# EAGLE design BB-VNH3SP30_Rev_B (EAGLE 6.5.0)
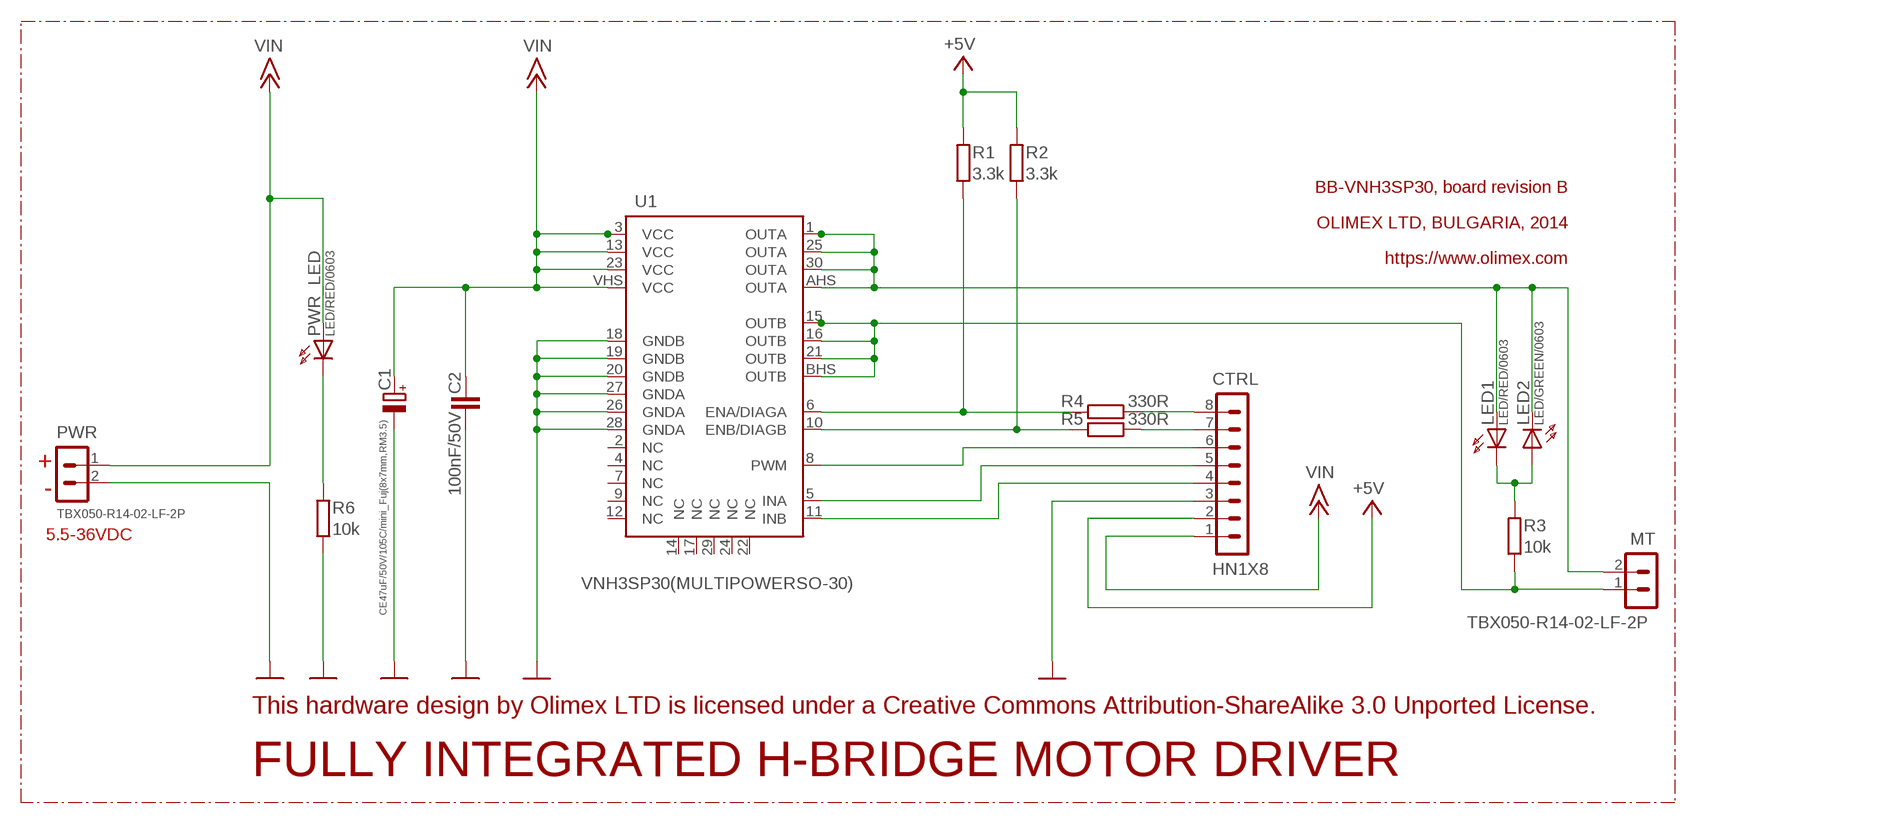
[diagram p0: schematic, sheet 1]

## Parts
C1  CE47uF/50V/105C/mini_Fuj(8x7mm,RM3.5)  CPOL-EUE3.5-8  [E3,5-8]
C2  100nF/50V  C-EUC0603_DWS  [C0603_DWS]
CTRL  HN1X8  CON8HN1X8  [HN1X8]
LED1  LED/RED/0603  LED0603DWS  [LED-0603]
LED2  LED/GREEN/0603  LED0603DWS  [LED-0603]
MT  TBX050-R14-02-LF-2P  CON2_TBX050-R14-02-LF-2P  [TBX050-R14-02-LF-2P]
PWR  TBX050-R14-02-LF-2P  CON2_TBX050-R14-02-LF-2P  [TBX050-R14-02-LF-2P]
PWR_LED  LED/RED/0603  LED0603DWS  [LED-0603]
R1  3.3k  R-EU_R0603_5MIL_DWS  [R0603_5MIL_DWS]
R2  3.3k  R-EU_R0603_5MIL_DWS  [R0603_5MIL_DWS]
R3  10k  R-EU_R0603_5MIL_DWS  [R0603_5MIL_DWS]
R4  330R  R-EU_R0603_5MIL_DWS  [R0603_5MIL_DWS]
R5  330R  R-EU_R0603_5MIL_DWS  [R0603_5MIL_DWS]
R6  10k  R-EU_R0603_5MIL_DWS  [R0603_5MIL_DWS]
U1  VNH3SP30(MULTIPOWERSO-30)  [MULTIPOWERSO-30]

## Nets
+5V: CTRL.2 R1.2 R2.2
+15V: C1.+ C2.2 CTRL.1 PWR.1 PWR_LED.A U1.3(VCC) U1.13(VCC) U1.23(VCC) U1.VHS1 U1.VHS2 U1.VHS3 U1.VHS4 U1.VHS5 U1.VHS6 U1.VHS7 U1.VHS8 U1.VHS9 U1.VHS10 U1.VHS11 U1.VHS(VCC) ; supply symbol labelled VIN
GND [pwr]: C1.- C2.1 CTRL.3 PWR.2 R6.1 U1.18(GNDB) U1.19(GNDB) U1.20(GNDB) U1.26(GNDA) U1.27(GNDA) U1.28(GNDA)
N$1: R1.1 R4.2 U1.6(ENA/DIAGA)
N$2: LED1.C LED2.A R3.2
N$3: CTRL.8 R4.1
N$4: CTRL.7 R5.1
N$5: PWR_LED.C R6.2
N$9: CTRL.6 U1.8(PWM)
N$10: R2.1 R5.2 U1.10(ENB/DIAGB)
N$11: CTRL.5 U1.5(INA)
N$16: CTRL.4 U1.11(INB)
OUTA: LED1.A LED2.C MT.2 U1.1(OUTA) U1.25(OUTA) U1.30(OUTA) U1.AHS1 U1.AHS2 U1.AHS3 U1.AHS4 U1.AHS5 U1.AHS(OUTA)
OUTB: MT.1 R3.1 U1.15(OUTB) U1.16(OUTB) U1.21(OUTB) U1.BHS1 U1.BHS2 U1.BHS3 U1.BHS4 U1.BHS5 U1.BHS(OUTB)
Unconnected: U1.2(NC) U1.4(NC) U1.7(NC) U1.9(NC) U1.12(NC) U1.14(NC) U1.17(NC) U1.22(NC) U1.24(NC) U1.29(NC)

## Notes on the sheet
- BB-VNH3SP30, board revision B
- OLIMEX LTD, BULGARIA, 2014
- https://www.olimex.com
- +
- -
- 5.5-36VDC
- This hardware design by Olimex LTD is licensed under a Creative Commons Attribution-ShareAlike 3.0 Unported License.
- FULLY INTEGRATED H-BRIDGE MOTOR DRIVER

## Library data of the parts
C1 = rcl:CPOL-EU: POLARIZED CAPACITOR, European symbol
C2 = rcl:C-EU: CAPACITOR, European symbol
CTRL = Penko:CON8
LED1 LED2 PWR_LED = DOUBLE-SIDE:LED
MT PWR = Penko:CON2
R1-R6 = rcl:R-EU_: RESISTOR, European symbol
U1 = OLIMEX_IC:VNH3SP30: VNH3SP30 FULLY INTEGRATED H-BRIDGE MOTOR DRIVER

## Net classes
0 default: width 0.254 mm, drill 0.6 mm, clearance 0.254 mm
1 pwr: width 0.25 mm
2 thin: width 0.025 mm, clearance 0.025 mm
3 gsm_pwr: width 0.914 mm, drill 0.787 mm

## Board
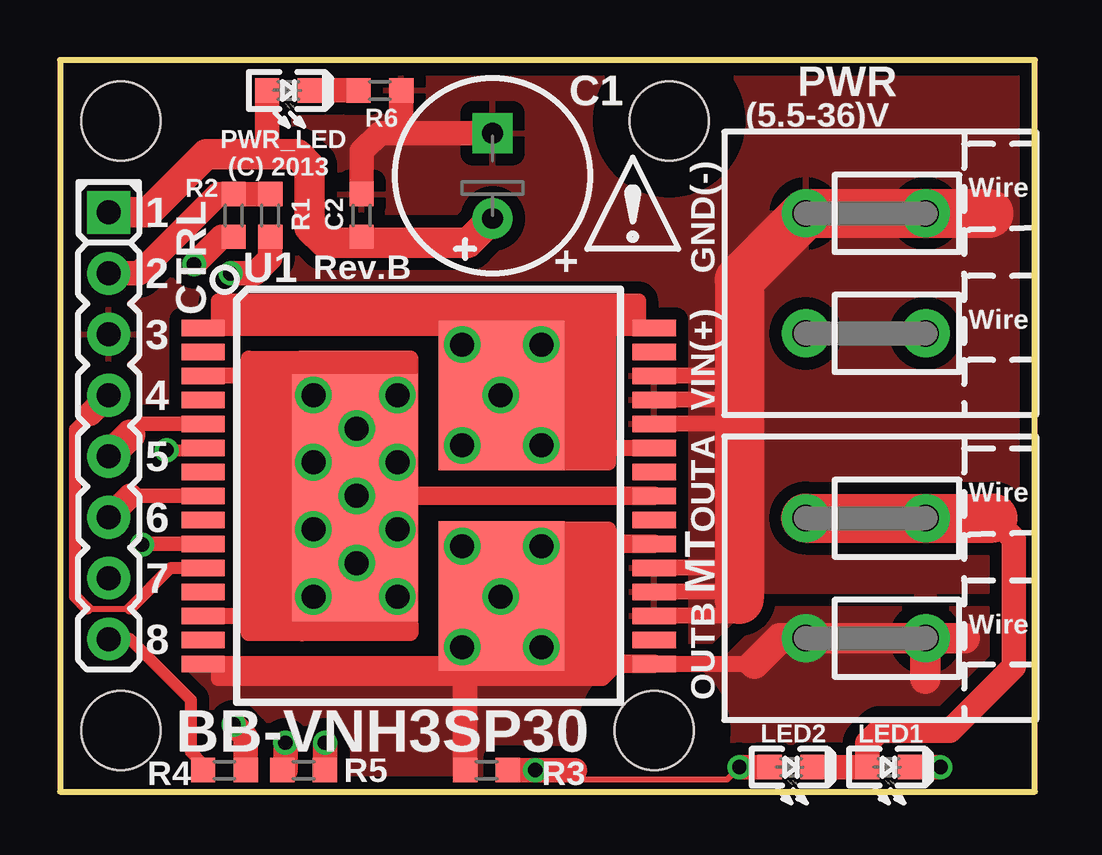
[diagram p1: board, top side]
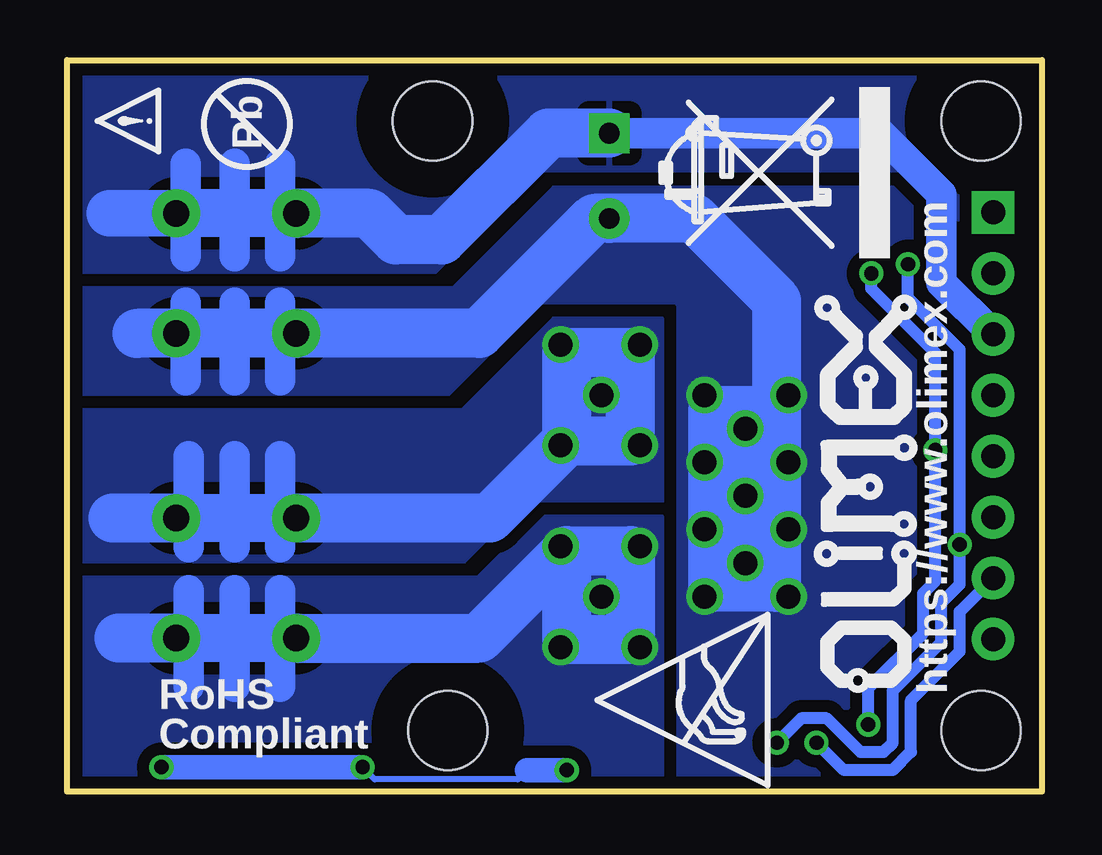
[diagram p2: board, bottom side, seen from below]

Size 40.64 x 30.48 mm. Coordinates in mm from the lower left corner, seen from the top.
Outline: 0,0 40.64,0 40.64,30.48 0,30.48 0,0
Copper layers (1+16): Top 0.035mm / dielectric 1.5mm / Bottom 0.035mm
Design rules "default": minimum track width 9.5mil, minimum drill 23mil, track to track 9.5mil, track to pad 9.5mil, pad to pad 9.5mil, via to via 10mil, smd to smd 1mil, copper to edge 10mil, drill to drill 8mil, minimum pad ring 10mil, minimum via ring 8mil, stop-mask expansion 4mil, vias tented up to drill 25mil, thermal gap 20mil
Holes 3.3 mm at 2.54,27.94 25.4,27.94 24.77,2.54 2.54,2.54
tRestrict: area 0,0 to 5.1,5.1; area 22.2,0 to 27.3,5.1; area 22.9,25.4 to 27.9,30.5; area 0,25.4 to 5.1,30.5
bRestrict: area 0,25.4 to 5.1,30.5; area 22.9,25.4 to 27.9,30.5; area 0,0 to 5.1,5.1; area 22.2,0 to 27.3,5.1

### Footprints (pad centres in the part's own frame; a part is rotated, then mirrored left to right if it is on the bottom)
E3,5-8 = drill 0.864 pad 1.676: + -1.778,0 | drill 0.864 pad 1.676 square: - 1.778,0
C0603_DWS = smd 1.016 x 1.016: 1 -0.889,0; 2 0.889,0
HN1X8 = drill 1 pad 1.778 square: 1 -8.89,0 | drill 1 pad 1.778: 2 -6.35,0; 3 -3.81,0; 4 -1.27,0; 5 1.27,0; 6 3.81,0; 7 6.35,0; 8 8.89,0
LED-0603 = smd 1.016 x 1.016: A 0.889,0; C -0.889,0
TBX050-R14-02-LF-2P = drill 1.1 pad 2: 1 -2.5,3.2; 2 2.5,3.2; 3 -2.5,-1.8; 4 2.5,-1.8
R0603_5MIL_DWS = smd 1.016 x 1.016: 1 -0.889,0; 2 0.889,0
MULTIPOWERSO-30 = smd 0.68 x 1.8: 1 -7,-9.4; 2 -6,-9.4; 3 -5,-9.4; 4 -4,-9.4; 5 -3,-9.4; 6 -2,-9.4; 7 -1,-9.4; 8 0,-9.4; 9 1,-9.4; 10 2,-9.4; 11 3,-9.4; 12 4,-9.4; 13 5,-9.4; 14 6,-9.4; 15 7,-9.4; 16 7,9.4; 17 6,9.4; 18 5,9.4; 19 4,9.4; 20 3,9.4; 21 2,9.4; 22 1,9.4; 23 0,9.4; 24 -1,9.4; 25 -2,9.4; 26 -3,9.4; 27 -4,9.4; 28 -5,9.4; 29 -6,9.4; 30 -7,9.4 | smd 6.23 x 5.25: AHS -4.173,3.049; BHS 4.163,3.047 | drill 1 pad 1.524: AHS1 -6.3,4.7; AHS2 -4.2,3; AHS3 -2.1,4.7; AHS4 -6.3,1.4; AHS5 -2.1,1.4; BHS1 2.1,4.7; BHS2 4.2,3; BHS3 6.3,4.7; BHS4 2.1,1.4; BHS5 6.3,1.4; VHS1 -4.2,-1.3; VHS2 -1.4,-1.3; VHS3 1.4,-1.3; VHS4 4.2,-1.3; VHS5 -4.2,-4.8; VHS6 -1.4,-4.8; VHS7 1.4,-4.8; VHS8 4.2,-4.8; VHS9 -2.8,-3; VHS10 0,-3; VHS11 2.8,-3 | smd 10.3 x 5.25: VHS 0.075,-3.055

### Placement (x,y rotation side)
C1  18.03,25.65 90 top
C2  12.57,24 270 top
CTRL  2.03,15.24 270 top
LED1  34.54,1.02 180 top
LED2  30.48,1.02 180 top
MT  34.29,8.89 90 top
PWR  34.29,21.59 90 top
PWR_LED  9.53,29.21 180 top
R1  8.76,24 90 top
R2  7.24,24 90 top
R3  17.78,0.89 0 top
R4  6.86,0.89 0 top
R5  10.16,0.89 0 top
R6  13.34,29.21 180 top
U1  15.37,12.32 270 top
U$1  [RECYCLE_BIN1/6]  6.35,22.23 90 bottom
U$2  [ATTENTION_SMALL]  36.83,26.67 90 bottom
U$3  [PB_SMALL]  33.15,27.81 90 bottom
U$4  [ATTENTION]  21.97,22.61 0 top
U$5  [ESD_SYMBOL]  11.43,0.25 90 bottom
U$14  [OLIMEX1_V]  5.08,21.84 90 bottom

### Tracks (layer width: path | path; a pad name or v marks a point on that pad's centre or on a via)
+5V
  Top 1.016: CTRL.2 3.3,21.59 6.6,24.89 R2.2 R1.2
+15V
  Top 0.61: 12.45,12.32 U1.VHS10 12.31,12.32 U1.VHS
  Top 0.66: 12.19,17.32 U1.3 | 12.19,12.24 12.19,17.32 | 12.19,12.24 U1.VHS | U1.13 9.91,7.32 | 9.91,7.32 12.19,7.32 12.19,12.24 | 9.91,7.32 10.03,7.32 10.03,6.99 | 10.03,6.99 10.03,6.6 10.16,6.6 | 10.16,6.6 14.61,6.6 14.61,6.99 10.03,6.99 | 12.19,17.32 14.61,17.32 14.61,17.78 | 14.61,17.78 14.61,18.03 10.03,18.03 | 10.03,17.78 10.03,17.27 | 14.61,17.78 10.03,17.78 | 10.16,6.6 7.87,6.6 7.87,18.03 10.03,18.03 | 10.03,17.78 10.03,18.03 | 10.03,17.78 8.38,17.78 8.38,6.99 9.53,6.99 9.53,16.76 8.89,16.76 8.89,7.49
  Top 0.762: U1.VHS 12.62,12.24 12.7,12.32 U1.23
  Top 1.016: 12.57,22.86 C2.2 | 8.64,26.54 PWR_LED.A
  Top 1.27: C1.+ 17.02,22.86 12.57,22.86 11.05,22.86 10.41,23.5 10.41,26.04 9.91,26.54 8.64,26.54 6.1,26.54 3.68,24.13 CTRL.1
  Top 2.032: U1.VHS 12.31,15.87 12.32,15.88
  Bottom 1.27: 33.66,17.14 33.66,19.09 33.66,20.36 | 35.69,17.14 35.69,19.09 35.69,20.36 | 31.75,20.36 31.75,19.09 31.75,17.14
  Bottom 2.032: 11.05,15.88 11.05,20.45 14.48,23.88 C1.+ 18.67,23.88 23.45,19.09 PWR.1 31.75,19.09 33.66,19.09 35.69,19.09 37.72,19.09 | 11.05,15.88 13.72,15.88 | 13.72,15.88 13.72,13.46 12.32,12.06 12.32,9.91 13.72,8.51 | 11.05,15.88 11.05,8.51 13.72,8.51 | 13.72,8.51 13.72,15.88 | 13.72,15.88 12.19,14.35 12.19,13.21
  pour Bottom (isolate 0.508, rank 3, no thermals): 41.91,20.95 24.51,20.95 20.32,25.15 6.1,25.15 3.17,22.23 -1.91,22.23 -1.91,-1.27 15.24,-1.27 15.24,20.32 20.57,20.32 24.38,16.51 41.91,16.51
GND
  Top 0.66: U1.18 28.32,7.32 28.32,8 | 28.32,8.32 U1.19 | 28.32,9.32 U1.20 | 28.32,16.38 28.45,16.38 | U1.26 28.57,15.32 28.57,16.32 | 28.32,16.64 28.57,16.64 28.57,16.32 | 28.57,16.32 U1.27 | 28.32,17.4 28.57,17.4 28.57,17.32 U1.28
  Top 1.016: C2.1 12.57,26.67 13.34,27.43 14.22,27.43 | C1.- 14.22,27.43 | 14.22,27.43 R6.1
  Top 2.032: 28.32,8 28.32,8.32 28.32,9.32 28.32,16.38 28.32,16.64 28.32,17.4 28.32,21.32 PWR.2 38.73,24.09
  Bottom 1.27: CTRL.3 4.19,21.21 4.19,24.89 6.73,27.43 C1.- | 33.66,24.09 33.66,24.38 | 33.66,24.38 33.66,26.16 | 35.69,24.09 35.69,24.38 | 35.69,24.38 35.69,26.16 | 31.75,24.09 31.75,24.38 | 31.75,24.38 31.75,26.16 | 31.75,24.38 31.75,22.31 | 33.66,24.38 33.66,22.31 | 35.69,24.38 35.69,22.31
  Bottom 1.93: PWR.2 31.75,24.09 33.66,24.09 35.69,24.09 38.86,24.09
  Bottom 2.032: PWR.2 28.03,24.09 26.92,22.99 25.02,22.99 20.57,27.43 C1.-
  pour Top (isolate 0.508, rank 4): -3.17,32.38 42.55,32.38 42.55,-1.27 -3.17,-1.27
  pour Bottom (isolate 0.508, rank 4): -1.91,31.75 -1.91,22.86 2.54,22.86 5.59,25.91 21.08,25.91 25.4,21.59 41.91,21.59 41.91,31.75
N$1  (via drill 0.6)
  Top 0.508: v4.45,14.22 5.97,14.22 U1.6
  Top 1.016: v7.11,21.59 8.13,21.59 8.76,22.23 R1.1 | v7.24,2.79 7.75,2.29 R4.2
  Bottom 0.508: v7.11,21.59 7.11,20.95 4.45,18.29 v4.45,14.22 4.45,8.76 4.95,8.26 4.95,6.6 7.24,4.32 v7.24,2.79
N$2  (via drill 0.6)
  Top 0.254: 21.46,0.89 21.84,0.51 27.81,0.51 v28.32,1.02
  Top 1.016: v36.7,1.02 LED1.C | v28.32,1.02 LED2.A | R3.2 v19.81,0.89 21.46,0.89
  Bottom 0.254: v28.32,1.02 27.81,0.51 21.84,0.51 21.46,0.89
  Bottom 1.016: v28.32,1.02 v36.7,1.02 | v19.81,0.89 21.46,0.89
N$3
  Top 0.508: CTRL.8 2.92,6.35 5.46,3.81 5.46,1.65 5.97,1.14 R4.1
N$4  (via drill 0.6)
  Top 1.016: v9.4,2.03 9.4,0.89 R5.1
  Bottom 0.508: CTRL.7 3.43,7.49 3.43,5.84 5.46,3.81 5.46,1.65 6.22,0.89 8.26,0.89 v9.4,2.03
N$5
  Top 1.016: R6.2 PWR_LED.C
N$9
  Top 0.61: 2.92,12.32 U1.8
  Top 1.016: CTRL.6 2.92,12.32
N$10  (via drill 0.6)
  Top 0.508: v3.43,10.29 3.46,10.32
  Top 0.61: 3.46,10.32 U1.10
  Top 1.016: v5.59,21.97 6.73,23.11 R2.1 | v11.05,2.03 R5.2
  Bottom 0.508: v5.59,21.97 5.59,20.57 3.43,18.41 v3.43,10.29 3.43,8.64 4.19,7.87 4.19,6.22 6.22,4.19 6.22,2.03 6.6,1.65 7.57,1.65 8.97,3.05 10.03,3.05 v11.05,2.03
N$11
  Top 0.61: 2.92,14.86 3.38,15.32 U1.5
  Top 1.27: CTRL.5 2.92,14.86
N$16
  Top 0.254: 1.14,7.62 2.92,7.62
  Top 0.508: 1.27,15.75 0.64,15.11 0.64,8.13 1.14,7.62 | U1.11 4.62,9.32 2.92,7.62
  Top 1.016: 1.27,15.75 CTRL.4
OUTA
  Top 0.61: 6.6,19.32 6.6,20.45 24.13,20.45 24.13,19.94 | 24.13,19.94 24.13,19.3 | 24.13,19.94 6.86,19.94 | U1.AHS 18.42,16.51 18.41,16.51 U1.AHS2
  Top 0.66: U1.1 6.6,19.32 18.41,19.32 | 18.41,19.32 U1.30 | 18.41,19.32 18.41,16.51 | 18.41,16.51 U1.AHS | 19.95,14.32 18.41,14.32 18.41,16.51 | 19.95,14.32 U1.25 | 19.95,14.32 19.95,13.72 22.86,13.72 22.86,19.18 21.21,19.18 21.21,14.73 22.35,14.73 22.35,18.8 21.84,18.8 21.84,15.24
  Top 1.016: LED2.C LED1.A 33.66,2.03 34.16,2.54 37.08,2.54 39.75,5.21 39.75,10.54 38.9,11.39
  Top 2.032: MT.2 38.9,11.39
  Bottom 1.27: MT.2 31.75,11.39 | 31.75,11.39 33.66,11.39 | 33.66,11.39 35.56,11.39 35.56,11.43 | 33.66,11.39 33.66,11.43 | 33.66,11.43 33.66,13.97 | 35.56,11.43 35.56,13.97 | 31.75,11.39 31.75,11.43 | 31.75,11.43 31.75,13.97 | 31.75,11.43 31.75,10.17 | 33.66,11.43 33.66,10.17 | 35.56,11.43 35.56,10.17
  Bottom 2.032: MT.2 23.03,11.39 19.81,14.61 17.14,14.61 17.14,18.29 19.81,18.29 19.81,14.73 | 35.56,11.39 38.73,11.39
  pour Bottom (isolate 0.508, rank 2, no thermals): 41.91,15.88 24.13,15.88 20.32,19.68 15.88,19.68 15.88,12.06 20.95,12.06 23.5,9.53 41.91,9.53
OUTB
  Top 0.61: 6.59,5.32 6.59,4.71 6.6,4.7 | 23.11,5.21 22.61,4.7 6.6,4.7 | 6.6,4.7 6.6,4.83 21.34,4.83
  Top 0.66: U1.BHS 18.41,8.38 | U1.BHS 18.41,8 | U1.15 6.59,5.32 18.41,5.32 18.41,8 | 18.41,8 U1.BHS | 18.41,8 16.89,6.48 | 20.57,10.03 20.57,10.92 22.86,10.92 22.86,5.97 | 22.86,5.97 22.86,5.46 | 22.86,5.97 21.21,5.97 21.21,9.65 22.48,9.65 22.48,6.6 21.72,6.6 21.72,9.14 22.1,9.14 22.1,6.99 22.23,6.99 | U1.16 28.94,5.32
  Top 0.762: U1.21 20.86,10.32 20.57,10.03 18.7,8.15 U1.BHS 18.39,8.15 | 18.39,8.15 18.29,8.26 | U1.16 21.22,5.32 18.39,8.15
  Top 1.016: 16.89,6.48 R3.1
  Top 1.27: 28.94,5.32 30.01,6.39 MT.1 36.07,6.39 | 36.07,6.39 37.72,6.39 | 36.07,6.39 36.07,4.7
  Bottom 1.27: MT.1 31.75,6.39 | 31.75,6.39 33.66,6.39 | 33.66,6.39 35.56,6.39 35.56,6.35 | 33.66,6.39 33.66,6.35 | 33.66,6.35 33.66,8.38 | 31.75,6.39 31.75,6.35 | 31.75,6.35 31.75,8.38 | 35.56,6.35 35.56,8.38 | 31.75,6.35 31.75,4.36 | 33.66,6.35 33.66,4.36 | 35.56,6.35 35.56,4.36
  Bottom 2.032: MT.1 23.45,6.39 19.81,10.03 | 19.81,10.03 17.14,10.03 17.14,6.35 19.81,6.35 19.81,10.03 | 35.56,6.39 38.48,6.39
  pour Bottom (isolate 0.508, no thermals): 41.91,8.89 23.5,8.89 20.95,11.43 15.88,11.43 15.88,-0.64 41.91,-0.64
  pour Top (isolate 0.508, no thermals): -1.91,5.08 27.3,5.08 29.84,7.62 41.91,7.62 41.91,-1.27 -1.91,-1.27

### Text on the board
tNames: (5.5-36)V | (C) 2013 | 1 | + | GND(-) | 2 | Rev.B | 3 | 4 | VIN(+) | 5 | 6 | OUTA | 7 | 8 | OUTB | BB-VNH3SP30
bNames: https://www.olimex.com | RoHS | Compliant
bStop: GND | VIN | OUTA | OUTB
